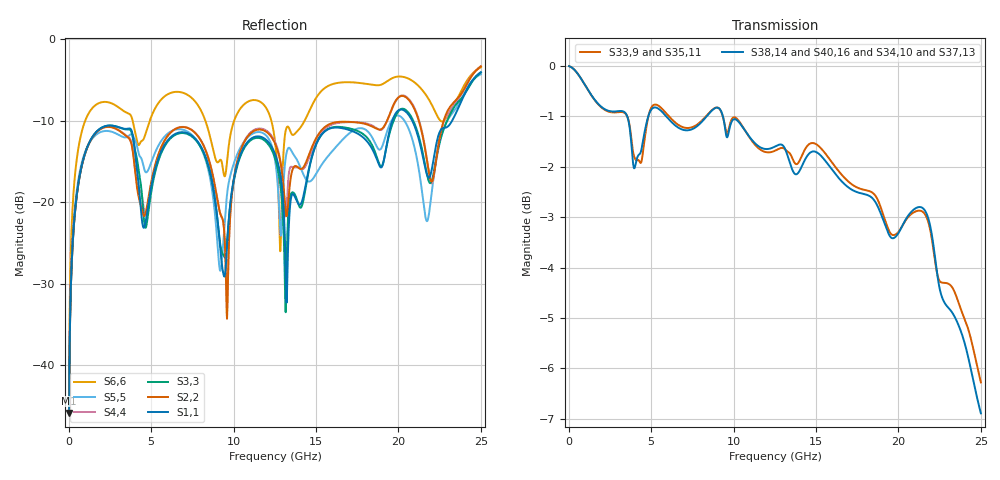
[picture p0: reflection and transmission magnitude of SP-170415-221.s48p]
! IMPORTANT NOTE: This model should not be used to evaluate
! electrical signals with a greater than 25 GHz. of frequency content.
! Please apply appropriate analysis techniques when reviewing the results of
! your simulations.
!  COPYRIGHT 2008, BY MOLEX INCORPORATED
!  ALL INTERNATIONAL RIGHTS RESERVED
!  THIS FILE CONTAINS MOLEX INCORPORATED CONFIDENTIAL INFORMATION
! >>>>>>>>>>>>>>>>  USER AGREEMENT  <<<<<<<<<<<<<<<<<<<
! The information on this media is the property of MOLEX Incorporated
! and  has been provided to you free of charge. Molex does not
! guarantee that the information is error-free, nor does MOLEX  make
! any representations, warranty or guarantee that the information is
! accurate, correct, reliable or up-to-date. MOLEX expressly
! disclaims all implied warranties regarding this information,
! including but not limited to any implied  warranties of
! merchantability or fitness for a particular purpose. MOLEX does
! not warrant that the media will work correctly in your multi- user
! or network environment.
! MOLEX will in no case be liable for your use, or the results of
! your use, of the software and other information contained on this
! media or  any accompanying written materials.  IT IS YOUR
! RESPONSIBILITY TO VERIFY THE RESULTS OF YOUR USE OF THIS
! INFORMATION IN YOUR OWN PARTICULAR ENGINEERING AND PRODUCT
! ENVIRONMENT, AND YOU ASSUME THE ENTIRE RISK OF DOING SO OR
! FAILING TO DO SO.  In no event will MOLEX be liable for any
! direct, indirect, incidental or consequential damages arising from
! your use of, or your inability to use, software, product simulations
! and other information contained on this media or any accompanying
! written materials.
! This model has not been validated with empirical data.
! This model was solved using HFSS.  TDR results can run 5-8 ohms low
! Touchstone file from project AM-170415-8022_rev11_10Dec
! Exported from HFSS 15.0.0
! Terminal data exported
! Port[1] = B1_T1
! Port[2] = C1_T1
! Port[3] = E1_T1
! Port[4] = F1_T1
! Port[5] = H1_T1
! Port[6] = J1_T1
! Port[7] = A2_T1
! Port[8] = B2_T1
! Port[9] = D2_T1
! Port[10] = E2_T1
! Port[11] = G2_T1
! Port[12] = H2_T1
! Port[13] = B3_T1
! Port[14] = C3_T1
! Port[15] = E3_T1
! Port[16] = F3_T1
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# GHZ S MA R 50.000000
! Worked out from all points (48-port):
!   1250 points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, 20 MHz to 25 GHz, reference 50 ohm
!   strongest paths, dB at 20 MHz, 6.26 GHz, 12.52 GHz, 18.76 GHz, 25 GHz:
!     S38,14: 0.0, -1.1, -1.6, -2.8, -6.9
!     S40,16: 0.0, -1.1, -1.6, -2.8, -6.8
!     S34,10: 0.0, -1.2, -1.6, -2.8, -6.1
!     S33,9: 0.0, -1.1, -1.7, -2.7, -6.3
!     S35,11: 0.0, -1.1, -1.6, -2.7, -6.6
!     S37,13: 0.0, -1.2, -1.6, -2.9, -6.5
!   lowest |S11| = -45.8 dB at 20 MHz (marker M1), VSWR 1.01, Z = 50 + j0.51 ohm
!   |S11| at or under -10 dB: start of sweep to 19.63 GHz; 20.84 GHz to 23.25 GHz (2.418 GHz wide, 11 % of centre)
